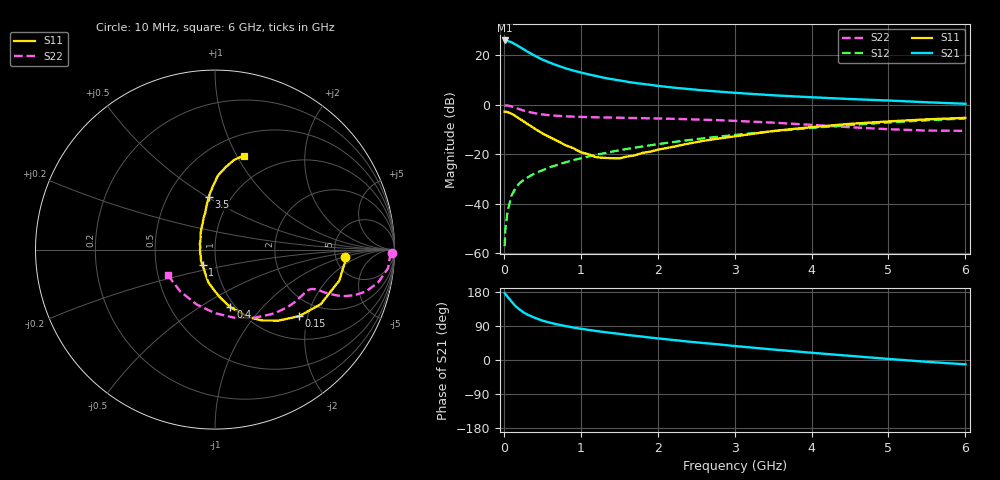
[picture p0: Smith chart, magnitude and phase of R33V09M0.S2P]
! SIEMENS Small Signal Semiconductors
! BFR181
! Si NPN RF Bipolar Junction Transistor in SOT23
! VCE = 3 V  IC = 9 mA
! Common Emitter S-Parameters:  May  1996
# GHz  S  MA  R  50
!  f  S11  S21  S12  S22
! GHz  MAG  ANG  MAG  ANG  MAG  ANG  MAG  ANG
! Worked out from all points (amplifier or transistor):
!   36 points, 10 MHz to 6 GHz, reference 50 ohm
!   highest |S21| = 26.0 dB at 10 MHz (marker M1)
!   |S21| within 3 dB of that: start of sweep to 227.1 MHz
!   unconditionally stable (mu >= 1): 794.1 MHz to 2.687 GHz
!   at 250 MHz: K = 0.58, MSG = 26.6 dB, |S12| = -30.5 dB
!   at 1.4 GHz: K = 1.06, MAG = 13.2 dB, |S12| = -18.9 dB
!   at 6 GHz: K = 0.85, MSG = 3.0 dB, |S12| = -5.5 dB
!   S11 on the Smith chart (normalised r, x): 10 MHz: 6.17, -1.03; 150 MHz: 1.53, -1.77; 400 MHz: 0.95, -0.68; 1 GHz: 0.86, -0.15; 3.5 GHz: 0.79, +0.51; 6 GHz: 0.71, +1.07
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0.01  0.7278 -3.1  20.02 177.0  0.0014 92.8  0.9857 -1.1
0.02  0.7273 -5.5  19.75 174.1  0.0031 83.4  0.9758 -2.4
0.05  0.7137 -14.0  19.53 166.5  0.0072 84.5  0.9694 -6.2
0.1  0.6631 -27.3  18.39 154.1  0.0147 76.4  0.9271 -11.4
0.15  0.598 -38.3  16.66 142.7  0.0205 73.2  0.8729 -15.5
0.2  0.5307 -48.2  15.04 133.9  0.0259 71.0  0.8204 -18.0
0.25  0.4722 -56.7  13.48 126.4  0.0298 68.2  0.7727 -19.6
0.3  0.4187 -63.6  12.05 120.5  0.0337 67.7  0.7341 -20.5
0.4  0.3328 -75.1  9.886 111.6  0.0413 67.2  0.6805 -21.2
0.5  0.2665 -84.2  8.24 103.9  0.0476 67.8  0.6423 -21.4
0.6  0.2222 -92.1  7.096 98.5  0.0552 68.3  0.6166 -21.3
0.7  0.1861 -101.3  6.221 93.8  0.0618 68.7  0.6003 -21.6
0.8  0.1536 -109.2  5.499 89.6  0.0689 68.7  0.5882 -21.9
1  0.1105 -128.9  4.505 82.5  0.0831 69.3  0.5715 -22.9
1.1  0.1006 -141.0  4.142 79.5  0.0905 69.5  0.5663 -23.5
1.3  0.0851 -164.1  3.54 73.9  0.1054 69.1  0.5567 -25.3
1.6  0.0904 159.1  2.939 66.2  0.1289 68.2  0.5462 -28.3
2.2  0.1422 121.7  2.235 52.9  0.1775 65.4  0.5231 -36.1
3.5  0.2967 96.8  1.562 27.7  0.2935 54.9  0.4378 -60.1
4.5  0.4141 87.6  1.313 10.9  0.3926 44.1  0.354 -90.1
5.5  0.5105 78.0  1.129 -4.8  0.4883 31.0  0.3028 -130.0
6  0.5467 73.1  1.053 -11.4  0.5311 23.9  0.299 -151.9
